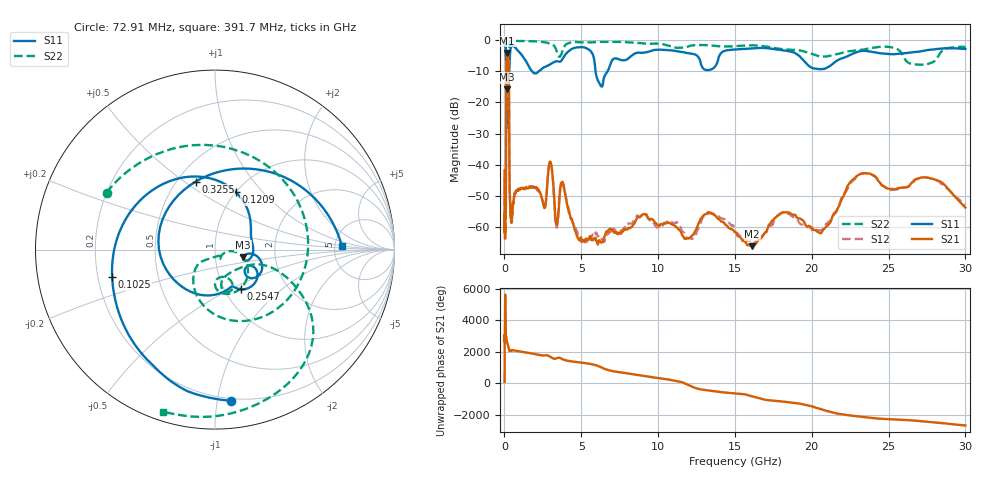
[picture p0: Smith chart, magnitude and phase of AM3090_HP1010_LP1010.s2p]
! Date/Time: Thu, Feb 28, 2019 2:04 PM
! Network Analyzer: Agilent Technologies E8364B Rev: A.07.50.67
! Sweep from 0.010 to 30.000 GHz, 1601 Points, Sweep Type: LOG
! Power Supply: 5.023 V, 0.002 A
# Hz S DB R 50
!freq MagS11 AngS11 MagS21 AngS21 MagS12 AngS12 MagS22 AngS22
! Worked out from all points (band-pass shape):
!   1601 points, 10 MHz to 30 GHz, reference 50 ohm
!   highest |S21| = -4.18 dB at 172.4 MHz (marker M1); lowest = -66.0 dB at 16.13 GHz (marker M2)
!   |S21| within 3 dB of the highest: 128 MHz to 274.2 MHz (146.1 MHz wide, 72.7 % of centre)
!   lowest |S11| = -15.8 dB at 156.8 MHz (marker M3), VSWR 1.39, Z = 68.2 - j6.15 ohm
!   |S11| at or under -10 dB: 122.1 MHz to 309.1 MHz (187 MHz wide, 86.7 % of centre); 1.792 GHz to 2.23 GHz (438.5 MHz wide, 21.8 % of centre); 5.927 GHz to 6.712 GHz (785.7 MHz wide, 12.4 % of centre)
!   |S22| runs from -28.3 to -0.2 dB; largest |S21 - S12| = 0.0096
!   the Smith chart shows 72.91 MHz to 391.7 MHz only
!   S11 on the Smith chart (normalised r, x): 72.91 MHz: 0.18, -1.09; 102.5 MHz: 0.26, -0.12; 120.9 MHz: 1.00, +0.72; 254.7 MHz: 1.19, -0.56; 325.5 MHz: 0.62, +0.55; 391.7 MHz: 5.79, +0.49
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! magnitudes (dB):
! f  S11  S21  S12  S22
! 10 MHz  -0.2  -41.7  -45.8  -0.7
! 38.04 MHz  -0.5  -59.5  -62.8  -1.5
! 72.91 MHz  -1.4  -53.6  -53.8  -3.3
! 102.5 MHz  -4.5  -37.5  -37.7  -5.6
! 120.9 MHz  -9.3  -11.5  -11.5  -11.9
! 144.7 MHz  -13.9  -4.8  -4.8  -25.3
! 156.8 MHz  -15.8  -4.3  -4.3  -22.4
! 172.4 MHz  -12.8  -4.2  -4.1  -13.8
! 254.7 MHz  -11.6  -5.5  -5.4  -12.5
! 287.2 MHz  -11.9  -11.0  -10.9  -10.7
! 325.5 MHz  -8.1  -44.7  -44.5  -1.3
! 391.7 MHz  -3.0  -55.1  -54.5  -0.5
! 550.5 MHz  -1.9  -52.4  -52.4  -0.3
! 2.084 GHz  -10.7  -47.3  -47.8  -0.5
! 2.987 GHz  -7.8  -38.9  -38.9  -1.2
! 3.385 GHz  -6.8  -59.3  -60.0  -3.4
! 3.779 GHz  -6.1  -45.6  -45.3  -3.4
! 5.077 GHz  -2.3  -64.3  -64.4  -0.7
! 7.926 GHz  -6.3  -60.6  -59.3  -0.7
! 16.13 GHz  -2.7  -66.0  -65.1  -1.7
! 23.24 GHz  -3.5  -42.8  -42.8  -3.2
! 30 GHz  -2.9  -53.7  -52.7  -2.2
